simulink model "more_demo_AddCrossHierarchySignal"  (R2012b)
settings: Solver=ode45  StartTime=0.0  StopTime=10.0  RelTol=1e-3

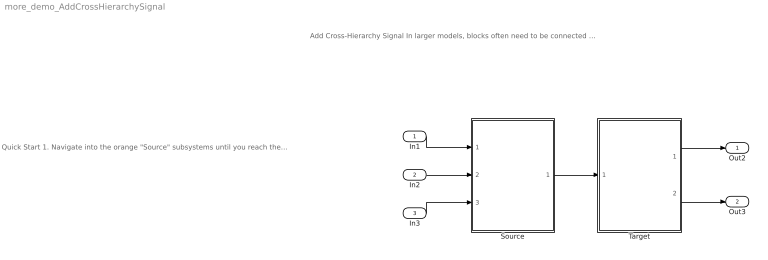
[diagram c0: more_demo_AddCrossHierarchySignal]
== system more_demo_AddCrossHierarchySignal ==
  note: Quick Start 1. Navigate into the orange "Source" subsystems until you reach the source block with a yellow background.
  note: Add Cross-Hierarchy Signal In larger models, blocks often need to be connected across multiple hierarchy levels. This action allows you to create signals between any blocks within the same model with just a few clicks.
  In1 : Inport
  In2 : Inport  Port=2
  In3 : Inport  Port=3
  Source : Subsystem
  Target : Subsystem
  Out2 : Outport
  Out3 : Outport  Port=2
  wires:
  Source/1(Out2) -> Target/1(In1)
  In1/1 -> Source/1(In1)
  In2/1 -> Source/2(In2)
  In3/1 -> Source/3(In3)
  Target/1(Out1) -> Out2/1
  Target/2(Out2) -> Out3/1

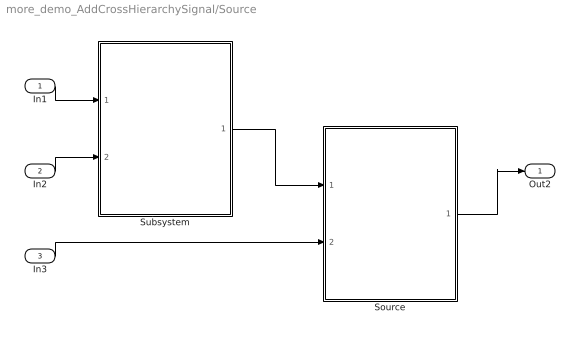
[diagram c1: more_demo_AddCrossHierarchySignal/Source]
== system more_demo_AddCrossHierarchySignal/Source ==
  In1 : Inport
  In2 : Inport  Port=2
  In3 : Inport  Port=3
  Source : Subsystem
  Subsystem : Subsystem
  Out2 : Outport
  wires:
  In1/1 -> Subsystem/1(In1)
  Source/1(Out1) -> Out2/1
  In2/1 -> Subsystem/2(In2)
  In3/1 -> Source/2(In2)
  Subsystem/1(Out1) -> Source/1(In1)

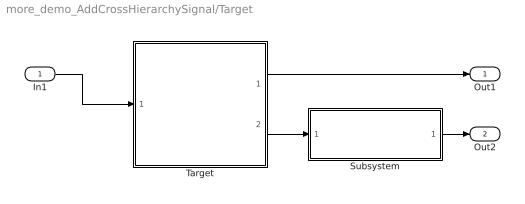
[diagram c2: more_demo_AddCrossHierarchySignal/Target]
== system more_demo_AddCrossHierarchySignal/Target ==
  In1 : Inport
  Subsystem : Subsystem
  Target : Subsystem
  Out1 : Outport
  Out2 : Outport  Port=2
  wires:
  Target/1(Out1) -> Out1/1
  Target/2(Out2) -> Subsystem/1(In1)
  Subsystem/1(Out1) -> Out2/1
  In1/1 -> Target/1(In1)

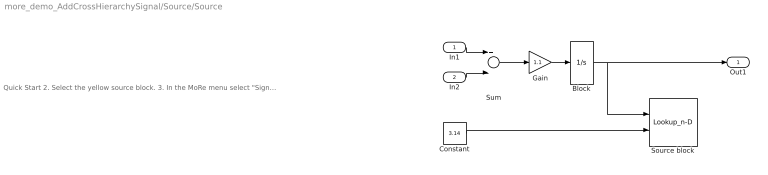
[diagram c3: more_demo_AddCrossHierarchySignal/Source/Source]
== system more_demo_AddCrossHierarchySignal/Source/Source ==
  note: Quick Start 2. Select the yellow source block. 3. In the MoRe menu select "Signal Routing -> Add Cross-Hierarchy Signal". 4. Leave the pop-up dialog open. To navigate to the target block, go back to the root level of this demo model and follow the green "Target" subsystems until you reach the target block highlighted in yellow.
  In1 : Inport
  In2 : Inport  Port=2
  Block : Integrator  InitialCondition=.589
  Constant : Constant  Value=3.14
  Gain : Gain  Gain=1.1
  Source block : Lookup_n-D  BreakpointsForDimension1=[1:3]  BreakpointsForDimension2=[1:3]  RndMeth=Simplest
  Sum : Sum  Inputs=+-
  Out1 : Outport
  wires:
  In2/1 -> Sum/2
  In1/1 -> Sum/1
  Gain/1 -> Block/1
  Constant/1 -> Source block/2
  Block/1 -> Source block/1, Out1/1
  Sum/1 -> Gain/1

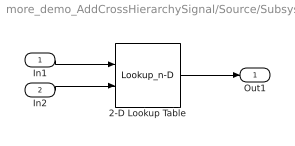
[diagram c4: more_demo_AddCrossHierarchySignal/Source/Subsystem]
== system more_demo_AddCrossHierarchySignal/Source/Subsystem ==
  In1 : Inport
  In2 : Inport  Port=2
  2-D Lookup Table : Lookup_n-D  BreakpointsForDimension1=[1:3]  BreakpointsForDimension2=[1:3]  RndMeth=Simplest
  Out1 : Outport
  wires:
  In1/1 -> 2-D Lookup Table/1
  In2/1 -> 2-D Lookup Table/2
  2-D Lookup Table/1 -> Out1/1

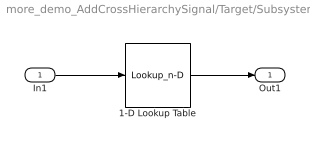
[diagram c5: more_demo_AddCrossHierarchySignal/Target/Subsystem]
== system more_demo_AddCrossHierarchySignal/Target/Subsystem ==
  In1 : Inport
  1-D Lookup Table : Lookup_n-D  NumberOfTableDimensions=1  BreakpointsForDimension1=[-5:5]  Table=tanh([-5:5])  RndMeth=Simplest
  Out1 : Outport
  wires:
  In1/1 -> 1-D Lookup Table/1
  1-D Lookup Table/1 -> Out1/1

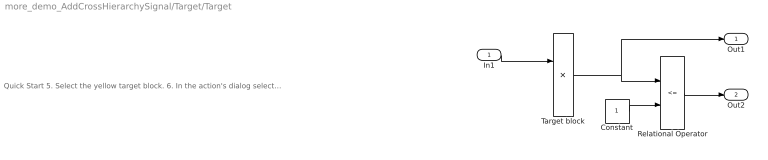
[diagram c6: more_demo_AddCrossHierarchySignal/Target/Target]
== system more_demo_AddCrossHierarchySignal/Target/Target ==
  note: Quick Start 5. Select the yellow target block. 6. In the action's dialog select "Get Selected Block". 7. In the "Name of Created Ports" you may specify a name for the ports that will be added by the action (e.g. "myAddedSignal"). 8. Select "Ok" and note the signal added to all levels from the source to the target block.
  In1 : Inport
  Constant : Constant
  Relational Operator : RelationalOperator  Operator=<=  OutDataTypeStr=boolean
  Target block : Product
  Out1 : Outport
  Out2 : Outport  Port=2
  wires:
  In1/1 -> Target block/1
  Target block/1 -> Out1/1, Relational Operator/1
  Relational Operator/1 -> Out2/1
  Constant/1 -> Relational Operator/2
